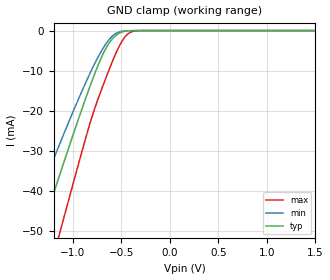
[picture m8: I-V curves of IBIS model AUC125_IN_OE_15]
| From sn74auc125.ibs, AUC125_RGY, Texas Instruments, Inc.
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[Model]   AUC125_IN_OE_15
Model_type  Input
Vinl=0.49
Vinh=1.04
| variable   typ   min   max
C_comp   2.61pF   2.18pF   3.00pF
[Temperature Range]   40   100   -40
| Ambient temperature   25   85   -40
[Voltage range]   1.5   1.4   1.6
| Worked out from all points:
|   GND clamp passes 1 mA (typ) near -0.55 V on its own axis
[GND Clamp]
| AUC125_IN_OE_15
|   Voltage   I(typ)   I(min)   I(max)
-3.6V     -222.6mA   -186.3mA   -267.8mA
-1.505V   -63.48mA   -50.79mA   -83.48mA
-1.325V   -49.98mA   -39.67mA   -67.42mA
-1.17V    -38.49mA   -30.3mA    -53.57mA
-1.12V    -34.83mA   -27.33mA   -49.09mA
-840mV    -14.99mA   -11.5mA    -24.46mA
-695mV    -6.117mA   -4.635mA   -14.06mA
-570mV    -1.488mA   -916.7uA   -6.381mA
-495mV    -364.6uA   -180.3uA   -2.692mA
-430mV    -73.19uA   -35.01uA   -776.9uA
-280mV    -781.4nA   -559.2nA   -5.358uA
1.5V      174.7pA    267.7pA    181.1pA
